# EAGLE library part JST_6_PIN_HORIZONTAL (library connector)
JST 6 pin horizontal connector JST-SH type. Here is the connector we sell at SparkFun: name (XXX-00000) Datasheet It was used on these SparkFun products: name (XXX-00000) name (XXX-00000)
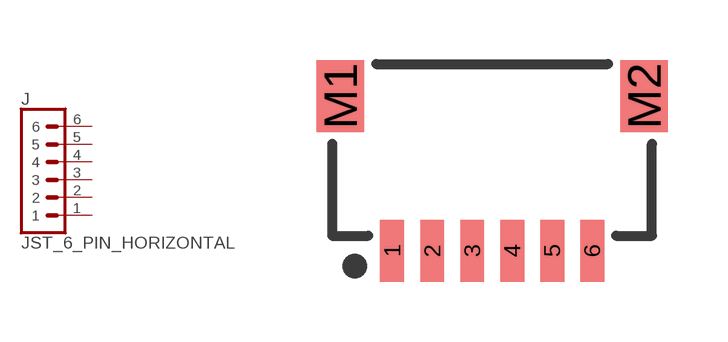
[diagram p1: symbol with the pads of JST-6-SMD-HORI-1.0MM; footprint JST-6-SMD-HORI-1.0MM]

Designator prefix J

## JST_6_PIN_HORIZONTAL (PROD_ID: XXX-00000; VALUE: BM06B-SRSS-TB)  [JST-6-SMD-HORI-1.0MM]
1  1  pas
2  2  pas
3  3  pas
4  4  pas
5  5  pas
6  6  pas

## Footprint JST-6-SMD-HORI-1.0MM (pad centres in mm)
JST SH Vertical 6-Pin SMT Specifications: Pin count:6 Pin pitch: 1 mm Datasheet referenced for footprint Example device(s): JST_6PIN_VERTICAL
smd 0.6 x 1.55: 1 -2.5,-4.775; 2 -1.5,-4.775; 3 -0.5,-4.775; 4 0.5,-4.775; 5 1.5,-4.775; 6 2.5,-4.775
smd 1.2 x 1.8: M1 -3.8,-0.9; M2 3.8,-0.9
